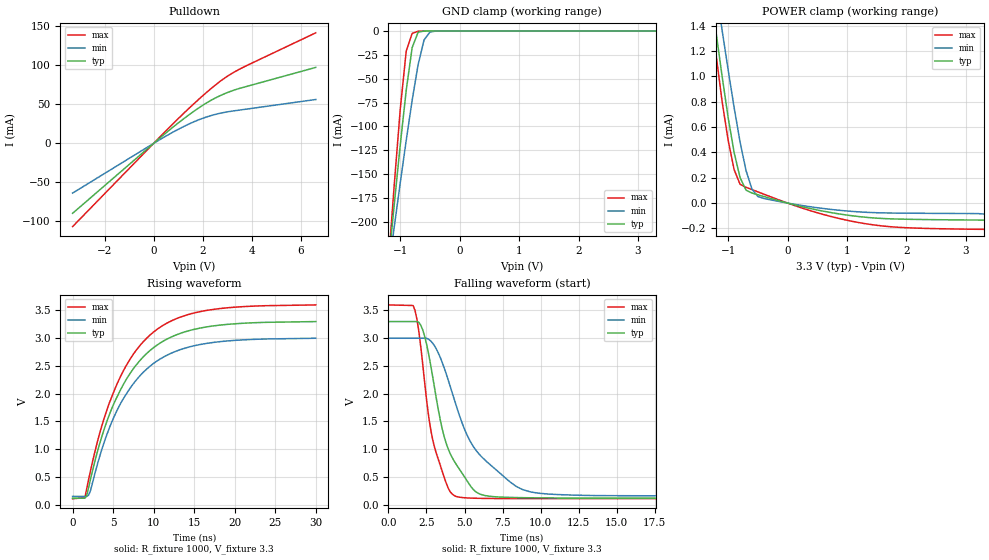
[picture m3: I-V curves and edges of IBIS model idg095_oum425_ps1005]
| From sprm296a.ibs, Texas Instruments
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[Model]   idg095_oum425_ps1005
Model_type   I/O_open_sink
Vinh = 2.00
Vinl = 0.80
Enable   Active-Low
Polarity   Non-Inverting
| signals   A, GZ, Y
Vmeas = 1.5
|   typ   min   max
C_comp   4.920p   4.867p   4.934p
|   typ   min   max
[Temperature Range]   25   -40   125
|   typ   min   max
[Voltage Range]   3.30V   3.00V   3.60V
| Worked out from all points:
|   slope of the pulldown table from 0 to 0.495 V, typ, clamps not added: 37.5 ohm
|   GND clamp passes 1 mA (typ) near -0.68 V on its own axis
|   POWER clamp passes 1 mA (typ) near -1.10 V on its own axis
|   falling waveform, R_fixture 1000, V_fixture 3.3: 20-80 % time 1.71ns typ, 2.98ns min, 1.19ns max; typ from 3.3 V to 0.117 V
|   rising waveform, R_fixture 1000, V_fixture 3.3: 20-80 % time 6.02ns typ, 5.99ns min, 5.99ns max; typ from 0.117 V to 3.3 V
[Pulldown]
|   Voltage   I(typ)   I(min)   I(max)
-3.3V     -89.53mA   -63.66mA   -106.5mA
600mV     15.94mA    11.1mA     19.19mA
1.5V      37.96mA    25.68mA    46.66mA
2.2V      52.64mA    34.23mA    66.46mA
2.8V      62.35mA    39.14mA    81.55mA
3.4V      69.44mA    42.18mA    93.31mA
6.6V      97.23mA    56.13mA    141.5mA
[GND_clamp]
|   Voltage   I(typ)   I(min)   I(max)
-3.3V     -1.677A    -1.286A    -2.145A
-1.2V     -245.1mA   -251.5mA   -244.4mA
-1.1V     -181.2mA   -204.9mA   -160.5mA
-1V       -119.5mA   -159.2mA   -82.09mA
-900mV    -62.33mA   -114.8mA   -21.2mA
-800mV    -17.44mA   -72.76mA   -2.57mA
-700mV    -1.313mA   -35.48mA   -250.1uA
-600mV    -54.63uA   -9.461mA   -14.12uA
-500mV    -2.522uA   -1.013mA   -487.5nA
-300mV    -4.308nA   -3.654uA   -305.3pA
3.3V      88.82pA    29.75nA    444.1pA
[POWER_clamp]
|   Voltage   I(typ)   I(min)   I(max)
-3.3V     9.016mA    8.661mA    9.714mA
-1.3V     1.684mA    1.994mA    1.543mA
-1.2V     1.335mA    1.674mA    1.159mA
-1.1V     995.1uA    1.359mA    796.1uA
-1V       674.2uA    1.051mA    495.5uA
-900mV    399.8uA    755.3uA    264.6uA
-800mV    201.5uA    482.5uA    148.7uA
-700mV    102.3uA    257.8uA    124.9uA
-600mV    79.32uA    110.4uA    106.6uA
-500mV    65.39uA    51.99uA    88.38uA
1.3V      -111.5uA   -72.32uA   -162.2uA
3.3V      -134.4uA   -86.65uA   -207.6uA
[Ramp]
|   I(typ)   I(min)   I(max)
dV/dt_r   0.001/20n   0.001/30n   0.001/10n
dV/dt_f   1.910/1.712n   1.710/2.975n   2.095/1.188n
[Falling Waveform]
R_fixture = 1000
V_fixture = 3.3
V_fixture_min = 3.0
V_fixture_max = 3.6
|  pd_on
|  TIME   V(typ)   V(min)   V(max)
0s        3.3V       3V         3.6V
1.752ns   3.3V       3V         3.5V
2.263ns   3.146V     3V         2.513V
2.646ns   2.712V     2.981V     1.589V
2.902ns   2.319V     2.913V     1.182V
3.669ns   1.222V     2.462V     492.3mV
4.436ns   735mV      1.803V     149.5mV
5.842ns   214.4mV    949.1mV    114.9mV
9.293ns   124.5mV    233.1mV    108.5mV
30ns      117.4mV    150.1mV    107.8mV
[Rising Waveform]
R_fixture = 1000
V_fixture = 3.3
V_fixture_min = 3.0
V_fixture_max = 3.6
|  pd_off
|  TIME   V(typ)   V(min)   V(max)
0s        117.4mV    149.9mV    107.8mV
1.505ns   117.4mV    149.9mV    124mV
1.971ns   306.4mV    170.9mV    451.7mV
3.603ns   1.226V     993.8mV    1.418V
5.468ns   1.936V     1.693V     2.168V
7.566ns   2.461V     2.191V     2.725V
9.897ns   2.816V     2.533V     3.097V
12.93ns   3.064V     2.772V     3.356V
16.66ns   3.203V     2.906V     3.5V
30ns      3.296V     2.996V     3.596V
